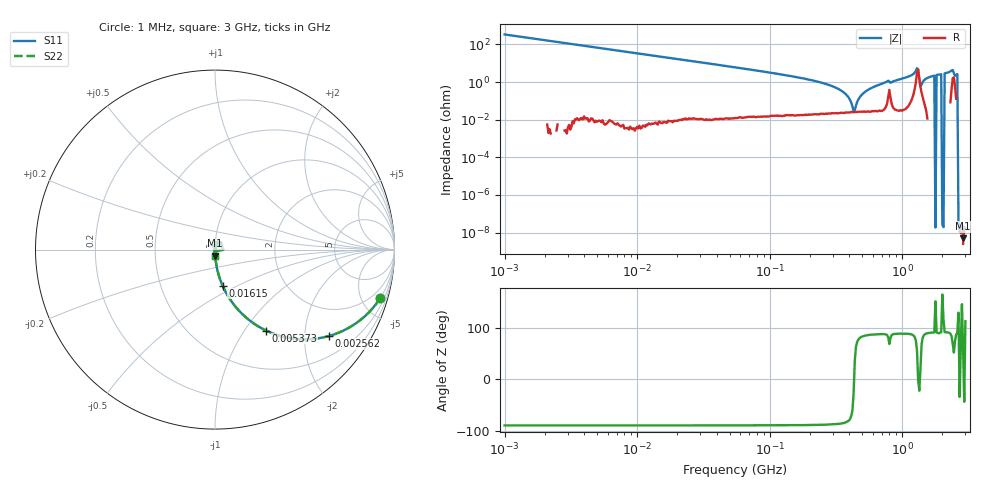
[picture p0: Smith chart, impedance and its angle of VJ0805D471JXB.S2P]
! VJ0805D471JXB
! DATE
! CORRECTED  DATA
# Hz  S  MA  R  50
!Freq	S11M	S11A	S21M	S21A	S12M	S12A	S22M	S22A
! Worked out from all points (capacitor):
!   401 points, 1 MHz to 3 GHz, reference 50 ohm
!   read as one part in series: C = 470 pF near 1.041 MHz
!   lowest |Z| = 4.97 nohm at 2.882 GHz (marker M1)
!   series resonance near 433.8 MHz, so ESL is about 290 pH
!   S11 on the Smith chart (normalised r, x): 1 MHz: 1.00, -6.78; 2.562 MHz: 1.00, -2.65; 5.373 MHz: 1.00, -1.26; 16.15 MHz: 1.00, -0.42; 3 GHz: 1.00, -0.07
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1000000  0.9592 -16.4  0.283 73.6  0.283 73.6  0.9592 -16.4
2561897  0.7977 -37.1  0.603 52.9  0.603 52.9  0.7977 -37.1
3823119  0.6633 -48.4  0.7483 41.6  0.7483 41.6  0.6633 -48.4
5372736  0.5334 -57.8  0.8458 32.2  0.8458 32.2  0.5334 -57.8
1.461624e7  0.2256 -76.9  0.9741 13.0  0.9741 13.0  0.2256 -76.9
1.615473e7  0.205 -78.1  0.9787 11.8  0.9787 11.8  0.205 -78.1
5.587962e7  0.05949 -86.5  0.9981 3.4  0.9981 3.4  0.05949 -86.5
2.094008e8  0.01238 -88.4  0.9997 0.7  0.9997 0.7  0.01238 -88.4
3.453811e8  0.003598 -86.1  0.9998 0.2  0.9998 0.2  0.003598 -86.1
3.894533e8  0.001705 -81.7  0.9998 0.1  0.9998 0.1  0.001705 -81.7
4.304467e8  0.0002782 -25.2  0.9997 0.0  0.9997 0.0  0.0002782 -25.2
4.853736e8  0.001793 81.4  0.9997 -0.1  0.9997 -0.1  0.001793 81.4
5.364635e8  0.003384 85.4  0.9997 -0.2  0.9997 -0.2  0.003384 85.4
8.005644e8  0.01051 68.1  0.9961 -0.6  0.9961 -0.6  0.01051 68.1
1.125055e9  0.02008 87.2  0.9992 -1.2  0.9992 -1.2  0.02008 87.2
1.268618e9  0.0391 73.4  0.9895 -2.2  0.9895 -2.2  0.0391 73.4
1.430499e9  0.01013 80.8  0.9984 -0.6  0.9984 -0.6  0.01013 80.8
1.581072e9  0.01762 89.0  0.9999 -1.0  0.9999 -1.0  0.01762 89.0
2.312676e9  0.037 86.6  0.9985 -2.1  0.9985 -2.1  0.037 86.6
2.556106e9  0.02406 85.6  0.9984 -1.4  0.9984 -1.4  0.02406 85.6
2.882277e9  0.0334 -87.1  1.002 -1.9  1.002 -1.9  0.0334 -87.1
3e9  0.0352 -87.1  1.002 -2.0  1.002 -2.0  0.0352 -87.1
